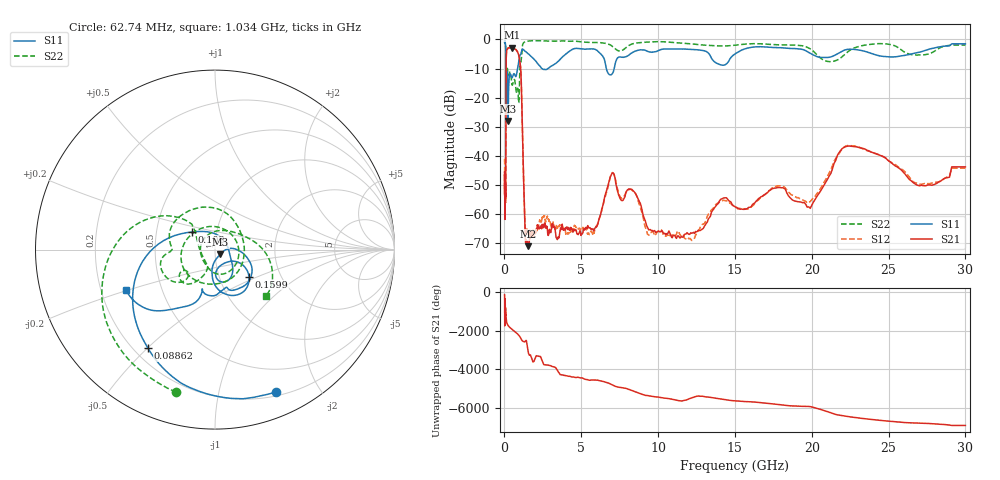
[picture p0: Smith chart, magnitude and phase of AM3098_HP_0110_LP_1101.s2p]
! Date/Time: Thu, Feb 28, 2019 8:38 AM
! Network Analyzer: Agilent Technologies E8364B Rev: A.07.50.67
! Sweep from 0.010 to 30.000 GHz, 1601 Points, Sweep Type: LOG
! Power Supply: 5.023 V, 0.002 A
# Hz S DB R 50
!freq MagS11 AngS11 MagS21 AngS21 MagS12 AngS12 MagS22 AngS22
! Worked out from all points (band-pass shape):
!   1601 points, 10 MHz to 30 GHz, reference 50 ohm
!   highest |S21| = -2.79 dB at 493.1 MHz (marker M1); lowest = -71.0 dB at 1.535 GHz (marker M2)
!   |S21| within 3 dB of the highest: 118.5 MHz to 944.7 MHz (826.2 MHz wide, 155 % of centre)
!   lowest |S11| = -28.0 dB at 237.5 MHz (marker M3), VSWR 1.08, Z = 53 - j2.78 ohm
!   |S11| at or under -10 dB: 99.92 MHz to 849.8 MHz (749.9 MHz wide, 158 % of centre); 2.448 GHz to 2.833 GHz (384.7 MHz wide, 14.6 % of centre); 6.631 GHz to 7.142 GHz (510.7 MHz wide, 7.42 % of centre)
!   |S22| runs from -22.2 to -0.4 dB; largest |S21 - S12| = 0.01
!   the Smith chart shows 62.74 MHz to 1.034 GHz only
!   S11 on the Smith chart (normalised r, x): 62.74 MHz: 0.24, -1.49; 88.62 MHz: 0.26, -0.50; 103 MHz: 0.76, +0.15; 159.9 MHz: 1.39, -0.44; 1.034 GHz: 0.31, -0.20
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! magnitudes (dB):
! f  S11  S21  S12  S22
! 10 MHz  -0.4  -46.5  -41.3  -0.6
! 38.04 MHz  -0.5  -60.2  -60.3  -1.0
! 62.74 MHz  -1.3  -51.4  -51.3  -1.7
! 88.62 MHz  -3.6  -42.8  -43.1  -3.9
! 103 MHz  -15.8  -14.0  -13.9  -20.1
! 144.7 MHz  -18.8  -3.9  -3.8  -14.0
! 159.9 MHz  -12.3  -3.6  -3.5  -11.4
! 237.5 MHz  -28.0  -3.0  -2.9  -12.1
! 493.1 MHz  -13.2  -2.8  -2.8  -15.6
! 550.5 MHz  -12.5  -3.0  -3.0  -15.0
! 926.3 MHz  -7.8  -5.4  -5.3  -21.7
! 1.034 GHz  -5.3  -8.9  -8.8  -8.3
! 1.328 GHz  -4.0  -64.4  -62.5  -0.8
! 1.535 GHz  -4.9  -71.0  -66.2  -0.6
! 2.084 GHz  -7.7  -65.2  -65.2  -0.5
! 5.612 GHz  -3.2  -65.1  -66.0  -1.0
! 6.959 GHz  -12.1  -46.4  -46.2  -2.1
! 7.926 GHz  -5.9  -52.3  -52.4  -2.7
! 11.95 GHz  -3.4  -66.7  -68.0  -1.4
! 19.8 GHz  -4.5  -57.5  -56.0  -2.9
! 22.56 GHz  -3.4  -36.7  -36.5  -3.5
! 30 GHz  -1.5  -43.7  -44.2  -1.9
